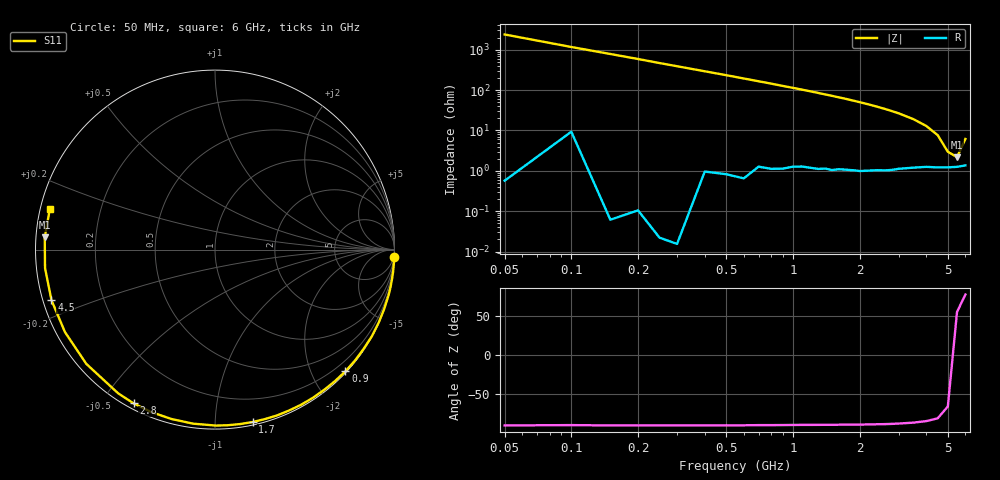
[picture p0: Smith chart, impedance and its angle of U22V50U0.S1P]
! SIEMENS Discrete & RF Semiconductors
! BBY52-02W
! Si Tuning Diode in SCD-80
! VR = 2.5 V
! S-Parameters:  September  1997
# GHz  S  MA  R  50
!  f  S11
! GHz  MAG  ANG
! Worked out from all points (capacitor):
!   34 points, 50 MHz to 6 GHz, reference 50 ohm
!   read as one part to ground: C = 1.35 pF near 50 MHz
!   lowest |Z| = 2.19 ohm at 5.5 GHz (marker M1)
!   series resonance near 5.301 GHz, so ESL is about 670 pH
!   S11 on the Smith chart (normalised r, x): 50 MHz: 0, -48; 900 MHz: 0.02, -2.54; 1.7 GHz: 0.02, -1.24; 2.8 GHz: 0.02, -0.60; 4.5 GHz: 0.02, -0.15; 6 GHz: 0.03, +0.12
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0.05  1 -2.4
0.2  1 -9.7
0.3  1 -14.6
0.4  0.9989 -19.4
0.5  0.9986 -24.1
0.6  0.9984 -28.9
0.8  0.9952 -38.3
0.9  0.9939 -43.0
1.1  0.9902 -52.0
1.2  0.9894 -56.5
1.3  0.9886 -60.9
1.4  0.9868 -65.3
1.5  0.9865 -69.5
1.6  0.9843 -73.7
1.7  0.9832 -77.7
1.8  0.9821 -81.8
2  0.9805 -89.7
2.2  0.9774 -97.2
2.4  0.9744 -104.4
2.6  0.9724 -111.3
2.8  0.9695 -117.9
3  0.9655 -124.0
3.5  0.9589 -138.4
4  0.954 -151.2
4.5  0.9536 -162.8
5  0.9525 -173.8
5.5  0.951 175.9
6  0.9476 166.3
